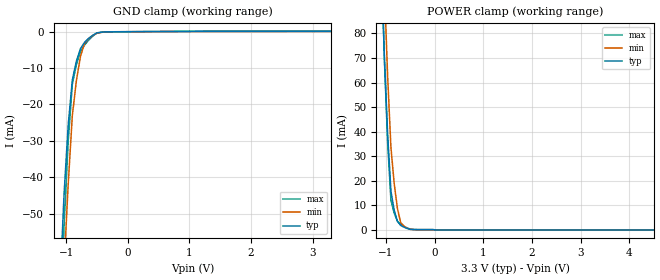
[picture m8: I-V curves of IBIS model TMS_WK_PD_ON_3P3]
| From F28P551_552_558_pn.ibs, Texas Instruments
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|   Model Cell TMS_WK_PD_ON_3P3
|TMS_WK_PD_ON_3P3
[Model]   TMS_WK_PD_ON_3P3
Model_type   Input
Polarity   Non-Inverting
Vinl =  0.8
Vinh =  2
C_comp   1.26765p   1.03155p   1.45072p
[Model Spec]
Vinl   0.8   0.8   0.8
Vinh   2   2   2
[Temperature Range]   25   155   -40
[Voltage Range]   3.3   2.97   3.63
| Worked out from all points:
|   GND clamp passes 1 mA (typ) near -0.57 V on its own axis
|   POWER clamp passes 1 mA (typ) near -0.61 V on its own axis
| Nom Voltages:
|   BIASFET=3.3, VDD=1.2, VDDS=3.3, VSS=0
| Min Voltages:
|   BIASFET=2.97, VDD=1.08, VDDS=2.97, VSS=0
| Max Voltages:
|   BIASFET=3.63, VDD=1.32, VDDS=3.63, VSS=0
[POWER_clamp]
|   voltage   I(typ)   I(min)   I(max)
-3.3V     1.919A     2.431A     2.069A
-1.1V     109.6mA    140.7mA    112.7mA
-1.033V   69.95mA    97.94mA    68.83mA
-966.7mV  38.69mA    62.25mA    35.3mA
-900mV    15.8mA     33.62mA    12.12mA
-833.3mV  8.097mA    18.99mA    6.857mA
-766.7mV  3.452mA    8.789mA    3.614mA
-700mV    1.864mA    3.003mA    2.391mA
-633.3mV  1.154mA    1.597mA    1.499mA
-500mV    241.1uA    272.7uA    323.7uA
-300mV    107.7uA    54.5uA     178.9uA
6.6V      0A         0A         0A
[GND_clamp]
|   voltage   I(typ)   I(min)   I(max)
-3.3V     -1.48A     -1.41A     -2.182A
-1.1V     -69.76mA   -89.94mA   -82.81mA
-1.033V   -44.5mA    -64.23mA   -52.88mA
-966.7mV  -25.67mA   -41.94mA   -30.09mA
-900mV    -13.26mA   -23.08mA   -14.45mA
-833.3mV  -8.078mA   -13.36mA   -9.007mA
-766.7mV  -4.616mA   -6.713mA   -5.399mA
-700mV    -2.875mA   -3.141mA   -3.626mA
-566.7mV  -946.7uA   -996.6uA   -1.185mA
-500mV    -315.3uA   -415.5uA   -372.2uA
-300mV    -28uA      -20.54uA   -40.77uA
3.3V      107.2uA    58.03uA    177.9uA
